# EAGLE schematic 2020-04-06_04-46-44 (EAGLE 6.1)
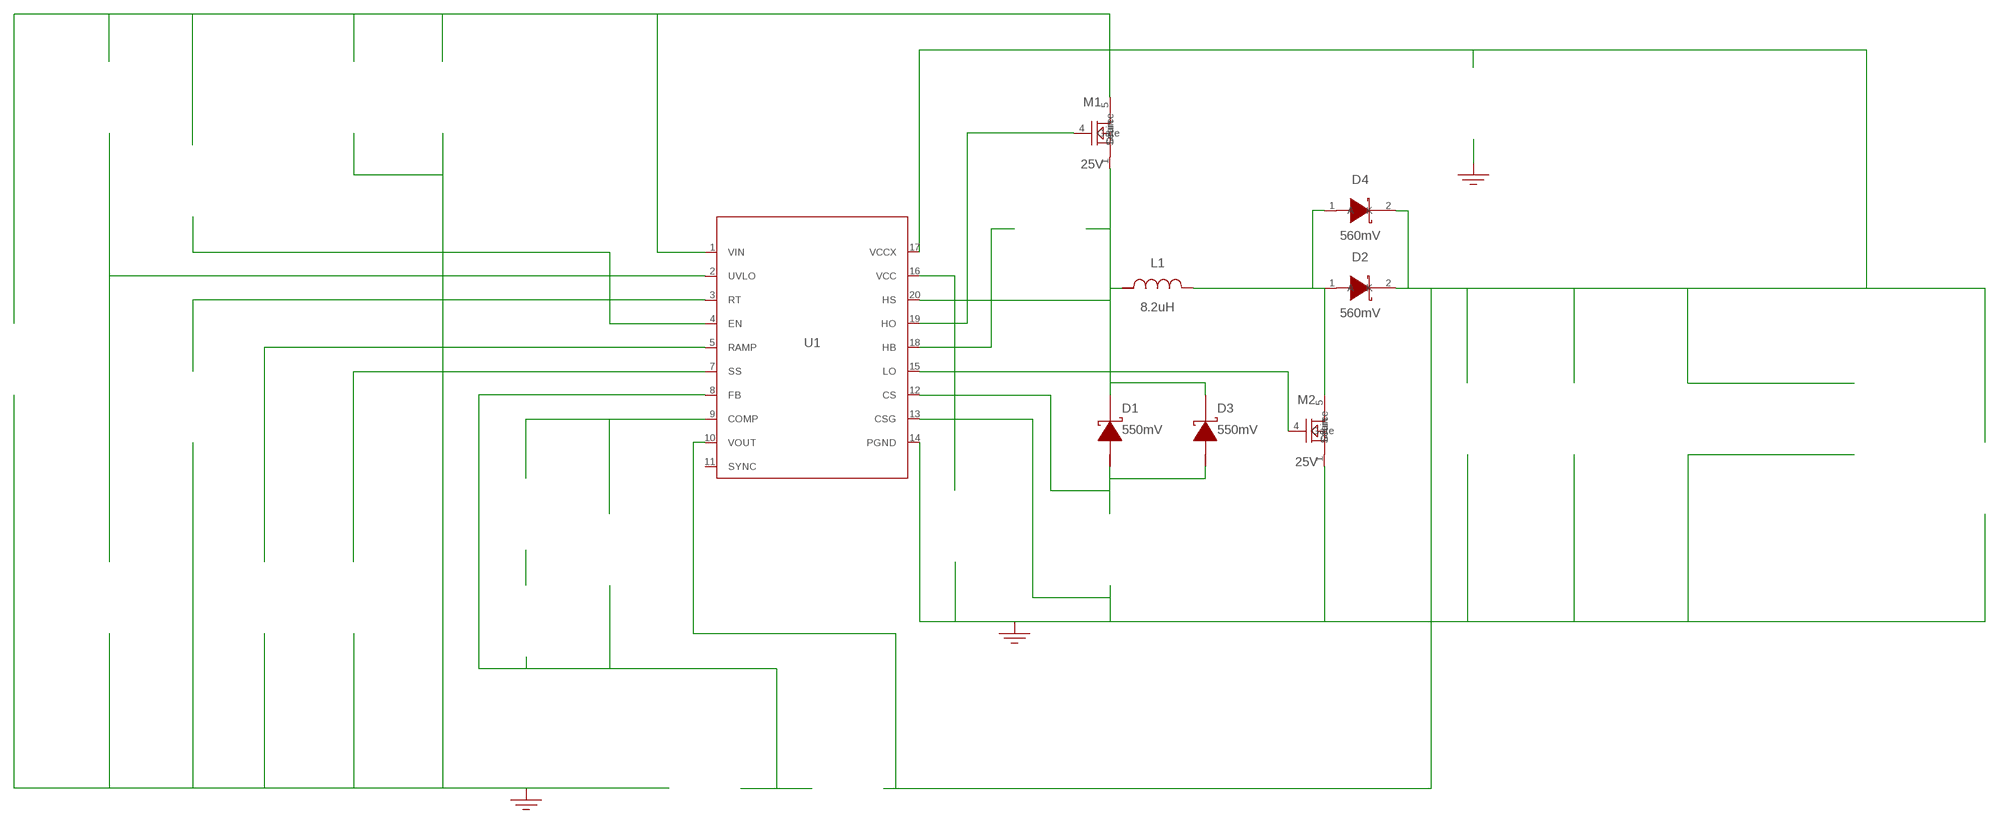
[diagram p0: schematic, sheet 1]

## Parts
CBOOT  100nF  08053C104JAZ2A08053C104JAZ2A  [0805]  (not placed on a sheet)
CCOMP  2.2nF  CL21C222JBFNNNECL21C222JBFNNNE  [0805]  (not placed on a sheet)
CCOMP2  100nF  08053C104JAZ2A08053C104JAZ2A  [0805]  (not placed on a sheet)
CIN  270uF  16SVPG270M16SVPG270M  [CAPSMT_62_C10]  (not placed on a sheet)
CINX  100nF  GRM155R71C104KA88DGRM155R71C104KA88D  [0402]  (not placed on a sheet)
COUT  560uF  20SVPF560M20SVPF560M  [CAPSMT_62_F12]  (not placed on a sheet)
COUT_2  560uF  20SVPF560M20SVPF560M  [CAPSMT_62_F12]  (not placed on a sheet)
COUT_3  560uF  20SVPF560M20SVPF560M  [CAPSMT_62_F12]  (not placed on a sheet)
COUTX  470nF  GRM155R61A474KE15DGRM155R61A474KE15D  [0402]  (not placed on a sheet)
COUTX2  470nF  GRM155R61A474KE15DGRM155R61A474KE15D  [0402]  (not placed on a sheet)
CRAMP  470pF  CL21C471KBANNNCCL21C471KBANNNC  [0805]  (not placed on a sheet)
CSS  22nF  CGA4J2C0G1H223J125AACGA4J2C0G1H223J125AA  [0805]  (not placed on a sheet)
CVCC  1uF  C0603C105Z8VACTUC0603C105Z8VACTU  [0603]  (not placed on a sheet)
CVCCX  1uF  C0603C105Z8VACTUC0603C105Z8VACTU  [0603]  (not placed on a sheet)
D1  550mV  B540C-13-FB540C-13-F  [SMC]
D2  560mV  PDS760-13PDS760-13  [PowerDI5]
D3  550mV  B540C-13-FB540C-13-F  [SMC]
D4  560mV  PDS760-13PDS760-13  [PowerDI5]
GND1  WB_GND  WB_GNDWB_GND  [WB_GND]
GND2  WB_GND  WB_GNDWB_GND  [WB_GND]
GND3  WB_GND  WB_GNDWB_GND  [WB_GND]
IOUT  WB_CURRENT_LOAD  WB_CURRENT_LOADWB_CURRENT_LOAD  [WB_CURRENT_LOAD]  (not placed on a sheet)
L1  8.2uH  7443735808274437358082  [WE-LHMI_8040]
M1  25V  CSD16340Q3CSD16340Q3  [DQG0008A]
M2  25V  CSD16340Q3CSD16340Q3  [DQG0008A]
RCOMP  12.1k  RC0201FR-0712K1LRC0201FR-0712K1L  [0201]  (not placed on a sheet)
RENABLE  1M  CRCW04021M00FKEDCRCW04021M00FKED  [0402]  (not placed on a sheet)
RFBB  1k  CRCW04021K00FKEDCRCW04021K00FKED  [0402]  (not placed on a sheet)
RFBT  3.05k  RT0805BRD073K05LRT0805BRD073K05L  [0805]  (not placed on a sheet)
RSENSE  10m  PMR100HZPFU10L0PMR100HZPFU10L0  [2512]  (not placed on a sheet)
RT  61.9k  CRCW040261K9FKEDCRCW040261K9FKED  [0402]  (not placed on a sheet)
RUV1  12.1k  RC0201FR-0712K1LRC0201FR-0712K1L  [0201]  (not placed on a sheet)
RUV2  12.1k  RC0201FR-0712K1LRC0201FR-0712K1L  [0201]  (not placed on a sheet)
U1  LM25118MH/NOPB  LM25118MH/NOPBLM25118MH/NOPB  [MXA20A]
VIN  WB_BATTERY  WB_BATTERYWB_BATTERY  [WB_BATTERY]  (not placed on a sheet)

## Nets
0: Cin.-@2 Cinx.2@2 Cout.-@2 Cout_2.-@2 Cout_3.-@2 Coutx2.2@2 Coutx.2@2 Cramp.2@2 Css.2@2 Cvcc.2@2 Cvccx.1@1 GND1.1 GND2.1 GND3.1 Iout.-@2 M2.1(Source) M2.2(Source) M2.3(Source) Rfbb.2@2 Rsense.2@2 Rt.2@2 Ruv2.2@2 U1.6(AGND) U1.13(CSG) U1.14(PGND) U1.21(EXP-PAD) Vin.-@2
1: Ruv1.2@2 Ruv2.1@1 U1.2(UVLO)
2: Rt.1@1 U1.3(RT)
3: Renable.2@2 U1.4(EN)
4: Cramp.1@1 U1.5(RAMP)
5: Css.1@1 U1.7(SS)
6: Cout.+@1 Cout_2.+@1 Cout_3.+@1 Coutx2.1@1 Coutx.1@1 Cvccx.2@2 D2.2(K) D4.2(K) Iout.+@1 Rfbt.1@1 U1.10(VOUT) U1.17(VCCX)
7: Ccomp2.2@2 Ccomp.2@2 Rfbb.1@1 Rfbt.2@2 U1.8(FB)
8: Ccomp.1@1 Rcomp.1@1 U1.9(COMP)
9: Cin.+@1 Cinx.1@1 M1.5(Drain) M1.6(Drain) M1.7(Drain) M1.8(Drain) M1.9(Drain) Renable.1@1 Ruv1.1@1 U1.1(VIN) Vin.+@1
10: Cboot.1@1 D1.1(K) D3.1(K) L1.2 M1.1(Source) M1.2(Source) M1.3(Source) U1.20(HS)
11: D1.2(A) D3.2(A) Rsense.1@1 U1.12(CS)
12: M2.4(Gate) U1.15(LO)
13: Ccomp2.1@1 Rcomp.2@2
14: Cvcc.1@1 U1.16(VCC)
15: M1.4(Gate) U1.19(HO)
16: Cboot.2@2 U1.18(HB)
17: D2.1(A) D2.3(A) D4.1(A) D4.3(A) L1.1 M2.5(Drain) M2.6(Drain) M2.7(Drain) M2.8(Drain) M2.9(Drain)
Unconnected: CBOOT.1 CBOOT.2 CCOMP2.1 CCOMP2.2 CCOMP.1 CCOMP.2 CIN.1(+) CIN.2(-) CINX.1 CINX.2 COUT.1(+) COUT.2(-) COUT_2.1(+) COUT_2.2(-) COUT_3.1(+) COUT_3.2(-) COUTX2.1 COUTX2.2 COUTX.1 COUTX.2 CRAMP.1 CRAMP.2 CSS.1 CSS.2 CVCC.1 CVCC.2 CVCCX.1 CVCCX.2 IOUT.1(+) IOUT.2(-) RCOMP.1 RCOMP.2 RENABLE.1 RENABLE.2 RFBB.1 RFBB.2 RFBT.1 RFBT.2 RSENSE.1 RSENSE.2 RT.1 RT.2 RUV1.1 RUV1.2 RUV2.1 RUV2.2 U1.11(SYNC) VIN.1(+) VIN.2(-)

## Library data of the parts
CBOOT CCOMP2 = AcceleratedDesigns_Lib:08053C104JAZ2A; Cap: 1.0E-7; Datasheet_URL: http://catalogs.avx.com/SurfaceMount.pdf; ESR: 0.0; IRMS: 0.0; Manufacturer_Name: AVX; Manufacturer_Part_Number: 08053C104JAZ2A; VDC: 25.0; Vendor: AVX
CCOMP = AcceleratedDesigns_Lib:CL21C222JBFNNNE; Cap: 2.2E-9; Datasheet_URL: http://www.samsungsem.com/servlet/FileDownload?type%3Dspec%26file%3DCL21C222JBFNNNE.pdf; ESR: 0.0; IRMS: 0.0; Manufacturer_Name: Samsung Electro-Mechanics; Manufacturer_Part_Number: CL21C222JBFNNNE; VDC: 50.0; Vendor: Samsung Electro-Mechanics
CIN = AcceleratedDesigns_Lib:16SVPG270M; Cap: 2.7E-4; Datasheet_URL: %20; ESR: 0.008; IRMS: 5.8; Manufacturer_Name: Panasonic; Manufacturer_Part_Number: 16SVPG270M; VDC: 16.0; Vendor: Panasonic
CINX = AcceleratedDesigns_Lib:GRM155R71C104KA88D; Cap: 1.0E-7; ESR: 0.0; IRMS: 0.0; Manufacturer_Name: MuRata; Manufacturer_Part_Number: GRM155R71C104KA88D; VDC: 16.0; Vendor: MuRata
COUT COUT_2 COUT_3 = AcceleratedDesigns_Lib:20SVPF560M; Cap: 5.6E-4; Datasheet_URL: http://industrial.panasonic.com/www%2Ddata/pdf/AAB8000/AAB8000CE1.pdf; ESR: 0.012; IRMS: 5.4; Manufacturer_Name: Panasonic; Manufacturer_Part_Number: 20SVPF560M; VDC: 20.0; Vendor: Panasonic
COUTX COUTX2 = AcceleratedDesigns_Lib:GRM155R61A474KE15D; Cap: 4.7E-7; ESR: 0.0; IRMS: 0.0; Manufacturer_Name: MuRata; Manufacturer_Part_Number: GRM155R61A474KE15D; VDC: 10.0; Vendor: MuRata
CRAMP = AcceleratedDesigns_Lib:CL21C471KBANNNC; Cap: 4.7E-10; Datasheet_URL: http://www.samsungsem.com/servlet/FileDownload?type%3Dspec%26file%3DCL21C471KBANNNC.pdf; ESR: 0.0; IRMS: 0.0; Manufacturer_Name: Samsung Electro-Mechanics; Manufacturer_Part_Number: CL21C471KBANNNC; VDC: 50.0; Vendor: Samsung Electro-Mechanics
CSS = AcceleratedDesigns_Lib:CGA4J2C0G1H223J125AA; Cap: 2.2E-8; Datasheet_URL: http://product.tdk.com/capacitor/mlcc/en/documents/mlcc%5Fautomotive%5Fgeneral%5Fen.pdf; ESR: 0.0; IRMS: 0.0; Manufacturer_Name: TDK; Manufacturer_Part_Number: CGA4J2C0G1H223J125AA; VDC: 50.0; Vendor: TDK
CVCC CVCCX = AcceleratedDesigns_Lib:C0603C105Z8VACTU; Cap: 1.0E-6; Datasheet_URL: http://www.kemet.com/kemet/web/homepage/kechome.nsf/vapubfiles/F3102%5FY5V.pdf/%24file/F3102%5FY5V.pdf; ESR: 0.001; IRMS: 0.0; Manufacturer_Name: Kemet; Manufacturer_Part_Number: C0603C105Z8VACTU; VDC: 10.0; Vendor: Kemet
D1 D3 = AcceleratedDesigns_Lib:B540C-13-F; Datasheet_URL: http://www.diodes.com/datasheets/ds13012.pdf; Io: 5.0; Manufacturer_Name: Diodes Inc.; Manufacturer_Part_Number: B540C-13-F; VFatIo: 0.55; VRRM: 40.0; Vendor: Diodes Inc.
D2 D4 = AcceleratedDesigns_Lib:PDS760-13; Datasheet_URL: www.diodes.com/datasheets/ds30477.pdf; Io: 7.0; Manufacturer_Name: Diodes Inc.; Manufacturer_Part_Number: PDS760-13; VFatIo: 0.56; VRRM: 60.0; Vendor: Diodes Inc.
GND1-GND3 = AcceleratedDesigns_Lib:WB_GND; Manufacturer_Name: WB_GND; Manufacturer_Part_Number: WB_GND; PowerPortType: POWER_GROUND; Value: Value
IOUT = AcceleratedDesigns_Lib:WB_CURRENT_LOAD; Manufacturer_Name: WB_CURRENT_LOAD; Manufacturer_Part_Number: WB_CURRENT_LOAD; PowerPortType: POWER_GROUND; Value: Value
L1 = AcceleratedDesigns_Lib:74437358082; DCR: 0.045; Datasheet_URL: http://katalog.we%2Donline.de/pbs/datasheet/74437358082.pdf; IDC: 13.0; L: 8.2E-6; Manufacturer_Name: Wurth Elektronik; Manufacturer_Part_Number: 74437358082; Vendor: Wurth Elektronik
M1 M2 = AcceleratedDesigns_Lib:CSD16340Q3; Datasheet_URL: http://www.ti.com/lit/ds/symlink/csd16340q3.pdf; IdsMax: 60.0; Manufacturer_Name: Texas Instruments; Manufacturer_Part_Number: CSD16340Q3; QgTyp: 6.5; Quantity: 1; Rdson45: 0.0043; VdsMax: 25.0; Vendor: Texas Instruments
RCOMP RUV1 RUV2 = AcceleratedDesigns_Lib:RC0201FR-0712K1L; Datasheet_URL: http://www.yageo.com/documents/recent/PYu%2DRC%5FGroup%5F51%5FRoHS%5FL%5F5.pdf; Manufacturer_Name: Yageo; Manufacturer_Part_Number: RC0201FR-0712K1L; Power: 0.05; Resistance: 12100.0; Tolerance: 1.0; Vendor: Yageo America
RENABLE = AcceleratedDesigns_Lib:CRCW04021M00FKED; Manufacturer_Name: Vishay-Dale; Manufacturer_Part_Number: CRCW04021M00FKED; Power: 0.063; Resistance: 1000000.0; Tolerance: 1.0; Vendor: Vishay-Dale
RFBB = AcceleratedDesigns_Lib:CRCW04021K00FKED; Manufacturer_Name: Vishay-Dale; Manufacturer_Part_Number: CRCW04021K00FKED; Power: 0.063; Resistance: 1000.0; Tolerance: 1.0; Vendor: Vishay-Dale
RFBT = AcceleratedDesigns_Lib:RT0805BRD073K05L; Manufacturer_Name: Yageo; Manufacturer_Part_Number: RT0805BRD073K05L; Power: 0.125; Resistance: 3050.0; Tolerance: 0.1; Vendor: Yageo America
RSENSE = AcceleratedDesigns_Lib:PMR100HZPFU10L0; Manufacturer_Name: Rohm; Manufacturer_Part_Number: PMR100HZPFU10L0; Power: 2.0; Resistance: 0.01; Tolerance: 1.0; Vendor: Rohm
RT = AcceleratedDesigns_Lib:CRCW040261K9FKED; Manufacturer_Name: Vishay-Dale; Manufacturer_Part_Number: CRCW040261K9FKED; Power: 0.063; Resistance: 61900.0; Tolerance: 1.0; Vendor: Vishay-Dale
U1 = AcceleratedDesigns_Lib:LM25118MH/NOPB; Datasheet_URL: http://www.ti.com/product/lm25118; Frequency: 500000.0; Imax: 20.0; Manufacturer_Name: Texas Instruments; Manufacturer_Part_Number: LM25118MH/NOPB; Mktg_Package: NA; NSID: LM25118MH/NOPB; Package: NA; Vendor: Texas Instruments
VIN = AcceleratedDesigns_Lib:WB_BATTERY; Manufacturer_Name: WB_BATTERY; Manufacturer_Part_Number: WB_BATTERY; PowerPortType: POWER_GROUND; Value: Value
